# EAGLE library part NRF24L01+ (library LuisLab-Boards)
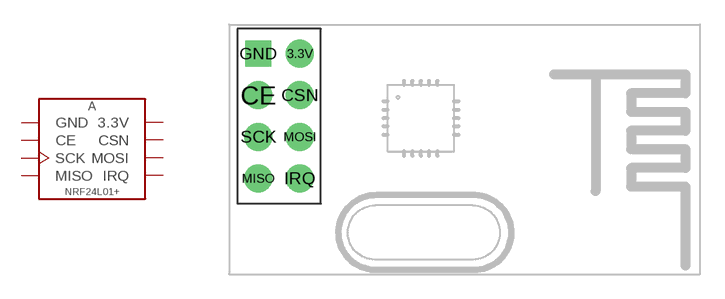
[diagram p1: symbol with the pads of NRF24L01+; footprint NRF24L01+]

Designator prefix A

## NRF24L01+  [NRF24L01+]
3.3V  3.3V
CE  CE
CSN  CSN
GND  GND
IRQ  IRQ
MISO  MISO
MOSI  MOSI
SCK  SCK

## Footprint NRF24L01+ (pad centres in mm)
drill 1.016 pad 1.7: 3.3V 1.27,3.81; CE -1.27,1.27; CSN 1.27,1.27; IRQ 1.27,-3.81; MISO -1.27,-3.81; MOSI 1.27,-1.27; SCK -1.27,-1.27
drill 1.016 pad 1.6 square: GND -1.27,3.81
